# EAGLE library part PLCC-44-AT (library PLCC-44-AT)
PLCC 44P THROUGH HOLE Source: Datasheet
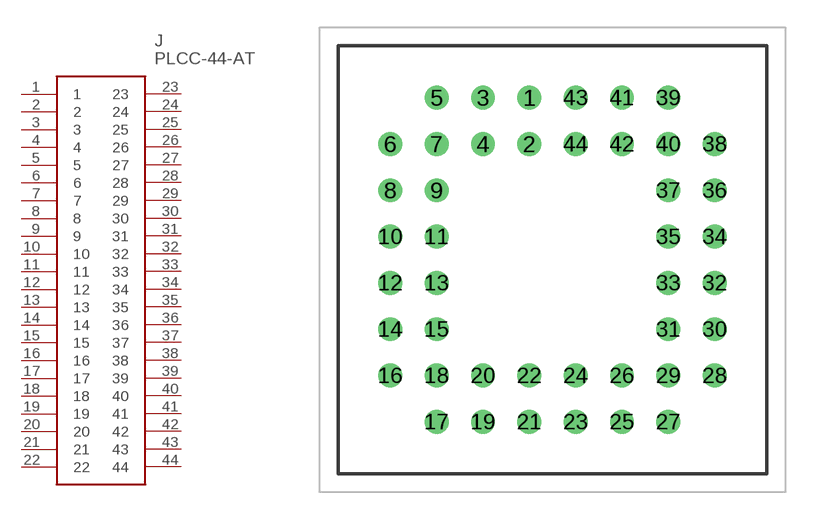
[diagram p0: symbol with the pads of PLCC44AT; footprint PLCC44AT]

Designator prefix J

## PLCC-44-AT (Arrow_Part_Number: PLCC-44-AT; Arrow_Price-Stock: https://www.arrow.com/en/products/plcc-44-at/adam-tech?region=nac; Description: PLCC 44P THROUGH HOLE; Height: 8.2mm; Manufacturer_Name: Adam Tech; Manufacturer_Part_Number: PLCC-44-AT)  [PLCC44AT]
1  1
2  2
3  3
4  4
5  5
6  6
7  7
8  8
9  9
10  10
11  11
12  12
13  13
14  14
15  15
16  16
17  17
18  18
19  19
20  20
21  21
22  22
23  23
24  24
25  25
26  26
27  27
28  28
29  29
30  30
31  31
32  32
33  33
34  34
35  35
36  36
37  37
38  38
39  39
40  40
41  41
42  42
43  43
44  44

## Footprint PLCC44AT (pad centres in mm)
23.5*23.5*8.2mm
drill 0.8 pad 1.3: 1 0,0; 2 0,-2.54; 3 -2.54,0; 4 -2.54,-2.54; 5 -5.08,0; 6 -7.62,-2.54; 7 -5.08,-2.54; 8 -7.62,-5.08; 9 -5.08,-5.08; 10 -7.62,-7.62; 11 -5.08,-7.62; 12 -7.62,-10.16; 13 -5.08,-10.16; 14 -7.62,-12.7; 15 -5.08,-12.7; 16 -7.62,-15.24; 17 -5.08,-17.78; 18 -5.08,-15.24; 19 -2.54,-17.78; 20 -2.54,-15.24; 21 0,-17.78; 22 0,-15.24; 23 2.54,-17.78; 24 2.54,-15.24; 25 5.08,-17.78; 26 5.08,-15.24; 27 7.62,-17.78; 28 10.16,-15.24; 29 7.62,-15.24; 30 10.16,-12.7; 31 7.62,-12.7; 32 10.16,-10.16; 33 7.62,-10.16; 34 10.16,-7.62; 35 7.62,-7.62; 36 10.16,-5.08; 37 7.62,-5.08; 38 10.16,-2.54; 39 7.62,0; 40 7.62,-2.54; 41 5.08,0; 42 5.08,-2.54; 43 2.54,0; 44 2.54,-2.54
